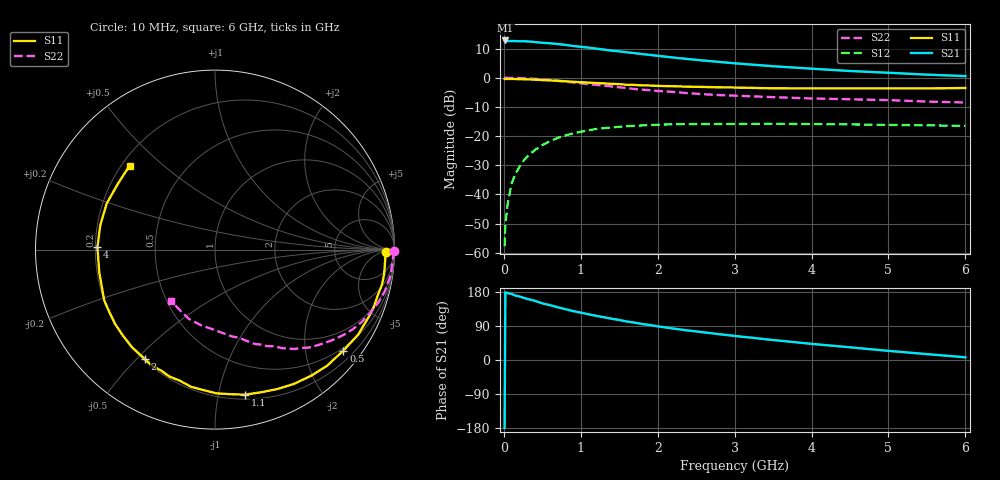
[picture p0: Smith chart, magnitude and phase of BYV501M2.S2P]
! SIEMENS Small Signal Semiconductors
! BFY420
! Si NPN RF SIEGET Grounded Emitter Transistor in MICRO-X
! VCE = 0.5 V  IC = 1.2 mA
! Common Emitter S-Parameters:  October  1996
# GHz  S  MA  R  50
!  f  S11  S21  S12  S22
! GHz  MAG  ANG  MAG  ANG  MAG  ANG  MAG  ANG
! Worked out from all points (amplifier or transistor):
!   36 points, 10 MHz to 6 GHz, reference 50 ohm
!   highest |S21| = 12.8 dB at 20 MHz (marker M1)
!   |S21| within 3 dB of that: start of sweep to 1.26 GHz
!   unconditionally stable (mu >= 1): 4.369 GHz to end of sweep
!   at 250 MHz: K = 0.05, MSG = 20.6 dB, |S12| = -28.7 dB
!   at 1.4 GHz: K = 0.27, MSG = 13.1 dB, |S12| = -17.0 dB
!   at 6 GHz: K = 1.33, MAG = 5.1 dB, |S12| = -16.5 dB
!   S11 on the Smith chart (normalised r, x): 10 MHz: 37, -12; 500 MHz: 0.43, -2.83; 1.1 GHz: 0.24, -1.20; 2 GHz: 0.21, -0.53; 4 GHz: 0.21, +0.01; 6 GHz: 0.23, +0.39
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0.01  0.9527 -0.9  4.326 -179.4  0.0013 88.1  0.9962 -0.5
0.02  0.9507 -1.8  4.347 178.6  0.003 86.2  0.9999 -0.9
0.05  0.9498 -4.1  4.243 176.4  0.007 86.9  0.9938 -2.3
0.1  0.9522 -8.1  4.25 174.3  0.0153 85.6  0.9907 -4.6
0.15  0.9507 -11.9  4.237 170.1  0.0224 81.7  0.9891 -7.1
0.3  0.9358 -23.3  4.192 161.4  0.0442 75.3  0.9743 -13.8
0.4  0.9276 -30.8  4.091 156.3  0.0573 70.2  0.9553 -18.2
0.5  0.9099 -38.2  3.962 149.5  0.07 65.7  0.9334 -22.4
0.7  0.884 -52.6  3.779 139.3  0.0928 56.8  0.8854 -30.2
0.8  0.8683 -59.4  3.649 134.2  0.1027 52.4  0.858 -33.8
0.9  0.8517 -65.7  3.5 129.1  0.1112 48.8  0.8299 -37.1
1.1  0.8251 -78.4  3.282 120.7  0.1258 41.6  0.7782 -43.4
1.4  0.7852 -94.7  2.906 108.9  0.1409 32.4  0.7096 -51.3
1.6  0.7562 -105.0  2.721 101.6  0.1481 27.4  0.6637 -55.8
2  0.7241 -122.7  2.374 88.8  0.1566 18.9  0.5933 -63.3
2.2  0.7139 -130.3  2.216 83.1  0.1592 14.9  0.5714 -67.0
2.8  0.6835 -149.7  1.863 68.1  0.1615 6.7  0.5034 -76.1
3.5  0.6571 -169.0  1.572 52.7  0.1627 -0.4  0.4642 -85.4
4  0.6551 178.9  1.428 42.6  0.1606 -4.6  0.441 -93.0
4.5  0.6535 167.9  1.303 33.5  0.1585 -8.5  0.4278 -100.9
5.5  0.6536 145.9  1.129 15.5  0.1526 -13.3  0.3906 -119.9
6  0.6671 135.5  1.065 7.1  0.1499 -14.1  0.3759 -130.9
